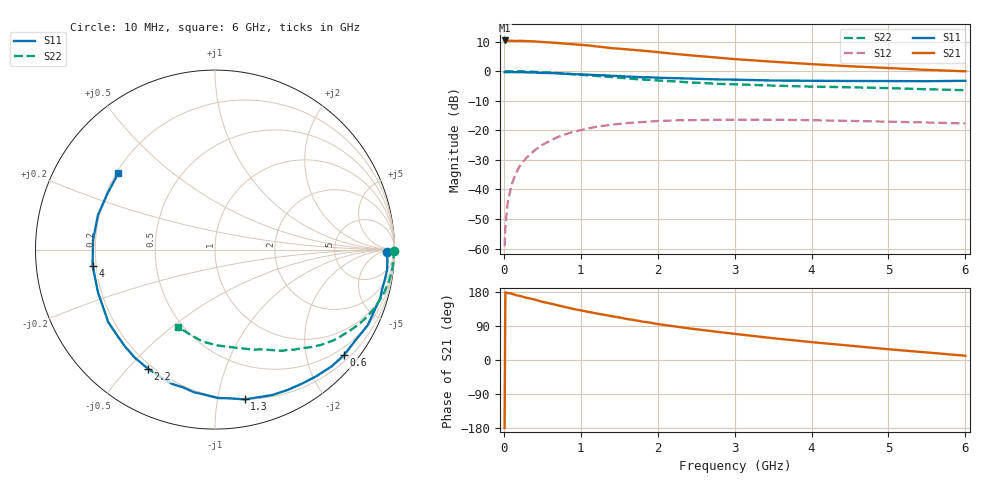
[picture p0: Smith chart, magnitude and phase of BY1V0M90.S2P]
! SIEMENS Small Signal Semiconductors
! BFY420
! Si NPN RF SIEGET Grounded Emitter Transistor in MICRO-X
! VCE = 1 V  IC = 0.9 mA
! Common Emitter S-Parameters:  October  1996
# GHz  S  MA  R  50
!  f  S11  S21  S12  S22
! GHz  MAG  ANG  MAG  ANG  MAG  ANG  MAG  ANG
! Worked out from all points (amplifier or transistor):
!   36 points, 10 MHz to 6 GHz, reference 50 ohm
!   highest |S21| = 10.4 dB at 10 MHz (marker M1)
!   |S21| within 3 dB of that: start of sweep to 1.593 GHz
!   unconditionally stable (mu >= 1): 4.582 GHz to end of sweep
!   at 250 MHz: K = 0.04, MSG = 20.4 dB, |S12| = -30.6 dB
!   at 1.4 GHz: K = 0.22, MSG = 13.0 dB, |S12| = -18.1 dB
!   at 6 GHz: K = 1.34, MAG = 5.3 dB, |S12| = -17.7 dB
!   S11 on the Smith chart (normalised r, x): 10 MHz: 43, -17; 600 MHz: 0.32, -2.77; 1.3 GHz: 0.20, -1.20; 2.2 GHz: 0.18, -0.57; 4 GHz: 0.19, -0.06; 6 GHz: 0.21, +0.33
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0.01  0.9608 -0.9  3.302 -179.3  0.0011 109.2  0.9999 -0.3
0.02  0.957 -1.3  3.274 178.7  0.0023 89.2  0.9915 -0.7
0.05  0.9624 -3.4  3.255 176.9  0.006 91.1  0.9971 -1.7
0.1  0.9657 -6.7  3.262 175.2  0.0119 85.5  0.9933 -3.6
0.15  0.961 -9.9  3.233 171.4  0.0179 84.0  0.9939 -5.3
0.25  0.9595 -16.5  3.244 166.7  0.0296 79.2  0.9876 -8.9
0.4  0.9496 -26.3  3.182 159.5  0.046 73.5  0.9734 -14.0
0.5  0.9319 -32.8  3.109 153.5  0.0566 69.3  0.9586 -17.4
0.6  0.9286 -39.3  3.056 149.2  0.0668 65.3  0.9441 -20.6
0.9  0.8903 -57.1  2.849 134.8  0.0939 54.0  0.8877 -29.5
1.1  0.8711 -68.4  2.72 127.0  0.108 47.3  0.8491 -34.9
1.3  0.8506 -78.8  2.54 119.4  0.1196 41.0  0.8109 -39.7
1.6  0.8103 -94.2  2.333 108.2  0.1325 32.8  0.7563 -46.1
1.8  0.7878 -103.0  2.217 101.4  0.1378 28.2  0.7235 -49.7
2.2  0.7616 -119.3  1.97 89.2  0.1468 19.4  0.6744 -56.8
2.4  0.75 -126.5  1.864 83.6  0.1484 16.1  0.6468 -60.0
2.8  0.7238 -139.5  1.685 73.7  0.1507 9.8  0.6096 -65.7
3.5  0.6941 -159.9  1.442 57.5  0.151 1.4  0.5704 -74.8
4  0.688 -172.6  1.314 47.2  0.1481 -3.4  0.5478 -81.8
4.5  0.6814 175.5  1.209 37.8  0.1442 -7.4  0.5336 -89.0
5.5  0.6758 152.2  1.05 19.9  0.1356 -12.2  0.494 -106.2
6  0.6867 141.6  0.995 11.2  0.1307 -12.6  0.4768 -115.9
